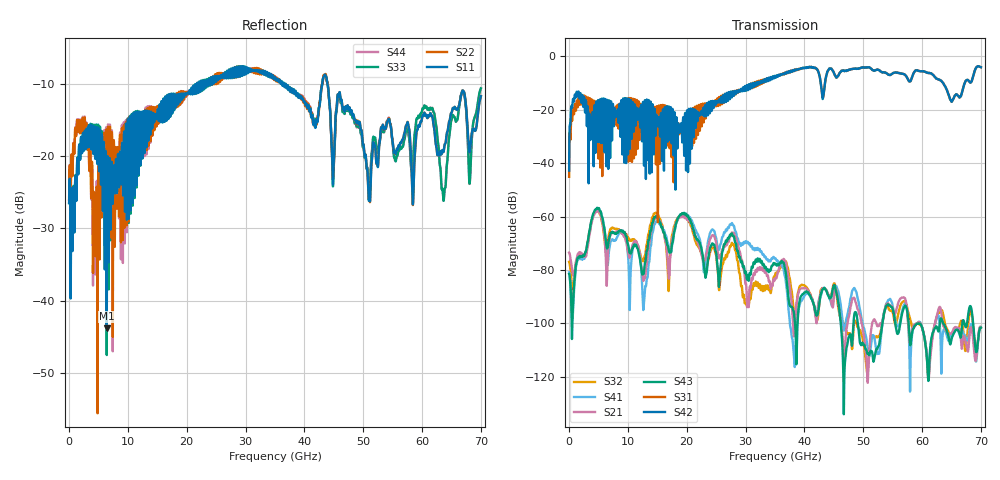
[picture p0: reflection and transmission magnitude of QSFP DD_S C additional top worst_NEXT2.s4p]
! AWR Design Environment (8415) Fri Dec 21 09:04:28 2018
! Document = 'CHANNEL TEST'
! nPorts: 4, nXvals: 7001
# HZ S DB R 50
!Freq DBS11 AngS11 DBS12 AngS12 DBS13 AngS13 DBS14 AngS14
!	DBS21 AngS21 DBS22 AngS22 DBS23 AngS23 DBS24 AngS24
!	DBS31 AngS31 DBS32 AngS32 DBS33 AngS33 DBS34 AngS34
!	DBS41 AngS41 DBS42 AngS42 DBS43 AngS43 DBS44 AngS44
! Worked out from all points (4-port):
!   7000 points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, 10 MHz to 70 GHz, reference 50 ohm
!   strongest paths, dB at 10 MHz, 17.51 GHz, 35.01 GHz, 52.51 GHz, 70 GHz:
!     S42: -42.7, -23.1, -7.5, -5.0, -4.0
!     S31: -45.1, -23.1, -7.6, -5.0, -4.0
!     S43: -81.5, -70.1, -77.8, -108.8, -101.5
!     S21: -73.5, -68.5, -83.3, -101.0, -101.5
!     S41: -80.8, -70.7, -75.6, -111.1, -101.4
!     S32: -76.9, -67.0, -82.0, -104.9, -101.6
!   lowest |S11| = -43.8 dB at 6.41 GHz (marker M1), VSWR 1.01, Z = 50.5 - j0.428 ohm
!   |S11| at or under -10 dB: start of sweep to 21.78 GHz; 36.52 GHz to 43.04 GHz (6.515 GHz wide, 16.4 % of centre); 43.91 GHz to end of sweep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
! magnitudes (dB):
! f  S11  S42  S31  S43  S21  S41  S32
! 10 MHz  -26.5  -42.7  -45.1  -81.5  -73.5  -80.8  -76.9
! 1.29 GHz  -24.2  -13.2  -16.8  -77.1  -75.7  -77.8  -76.5
! 4.79 GHz  -21.0  -31.6  -18.5  -56.7  -57.7  -56.9  -57.5
! 6.41 GHz  -43.8  -21.7  -18.7  -71.6  -85.6  -74.2  -73.1
! 19.28 GHz  -11.7  -29.4  -28.9  -58.7  -59.8  -58.8  -59.4
! 23.19 GHz  -9.8  -19.2  -23.1  -82.9  -75.4  -76.6  -78.6
! 70 GHz  -11.8  -4.0  -4.0  -101.5  -101.5  -101.4  -101.6
